(* Logix 5000 AddOnInstructionDefinition export TeNod4TBlocLegal; software revision 28.00 *)

ADD_ON_INSTRUCTION TeNod4TBlocLegal   (* revision 1.1, vendor Scaime *)
VAR_IN_OUT
   Datas : TeNod4TDatas; {required}
END_VAR
VAR_INPUT
   CaptureRead : BOOL; {visible}
   CaptureOnly : BOOL; {visible}
   RequestedID : DINT; {visible}
   Read : BOOL; {visible}
END_VAR
VAR_OUTPUT
   InProgress : BOOL; {visible}
   Done : BOOL; {visible}
   Error : BOOL; {visible}
   CapturedID : DINT; {access Read Only, visible}
END_VAR
VAR
   IntCapture1 : BOOL; {access None}
   IntCapture2 : BOOL; {access None}
   IntCapture3 : BOOL; {access None}
   ReadSeq : BOOL; {access None}
   ReadSeq1 : BOOL; {access None}
   ReadSeq2 : BOOL; {access None}
   ReadSeq3 : BOOL; {access None}
   ReadSeqDone : BOOL; {access None}
   IntRead1 : BOOL; {access None}
END_VAR

ROUTINE Logic   (* ladder *)
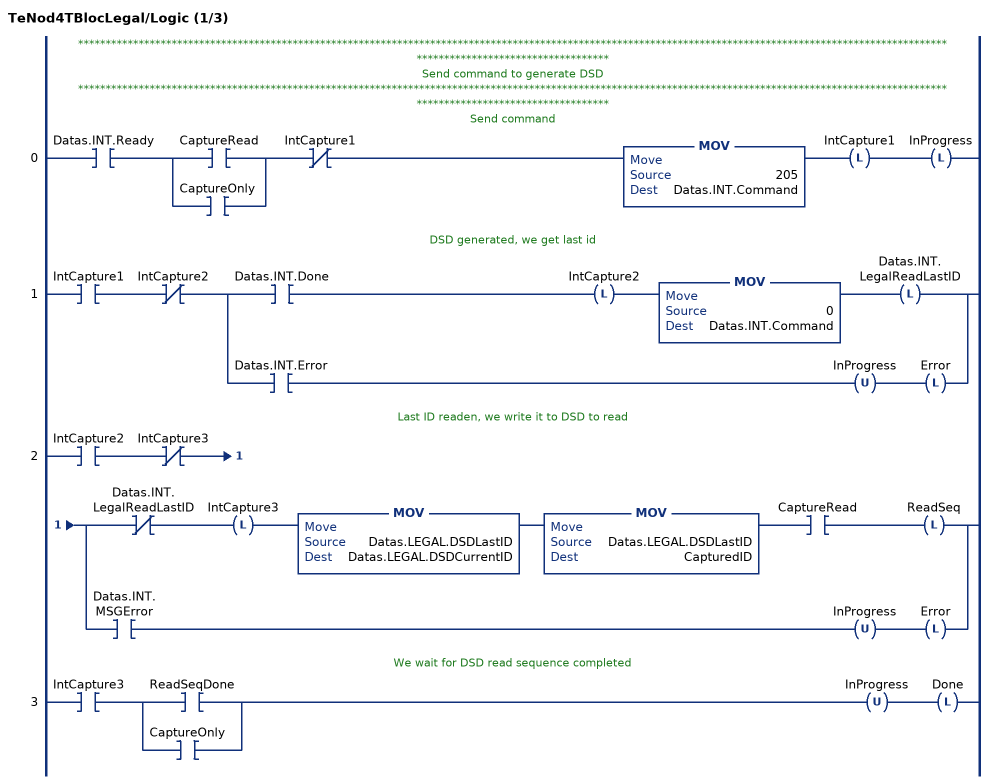
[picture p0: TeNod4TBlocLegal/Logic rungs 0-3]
   // *************************************************************************************************************************************************************************************************
   // Send command to generate DSD
   // *************************************************************************************************************************************************************************************************
   // Send command
   0: XIC(Datas.INT.Ready)[XIC(CaptureRead) ,XIC(CaptureOnly) ]XIO(IntCapture1)MOV(205,Datas.INT.Command)OTL(IntCapture1)OTL(InProgress);
   // DSD generated, we get last id
   1: XIC(IntCapture1)XIO(IntCapture2)[XIC(Datas.INT.Done) OTL(IntCapture2) MOV(0,Datas.INT.Command) OTL(Datas.INT.LegalReadLastID) ,XIC(Datas.INT.Error) OTU(InProgress) OTL(Error) ];
   // Last ID readen, we write it to DSD to read
   2: XIC(IntCapture2)XIO(IntCapture3)[XIO(Datas.INT.LegalReadLastID) OTL(IntCapture3) MOV(Datas.LEGAL.DSDLastID,Datas.LEGAL.DSDCurrentID) MOV(Datas.LEGAL.DSDLastID,CapturedID) XIC(CaptureRead) OTL(ReadSeq) ,XIC(Datas.INT.MSGError) OTU(InProgress) OTL(Error) ];
   // We wait for DSD read sequence completed
   3: XIC(IntCapture3)[XIC(ReadSeqDone) ,XIC(CaptureOnly) ]OTU(InProgress)OTL(Done);
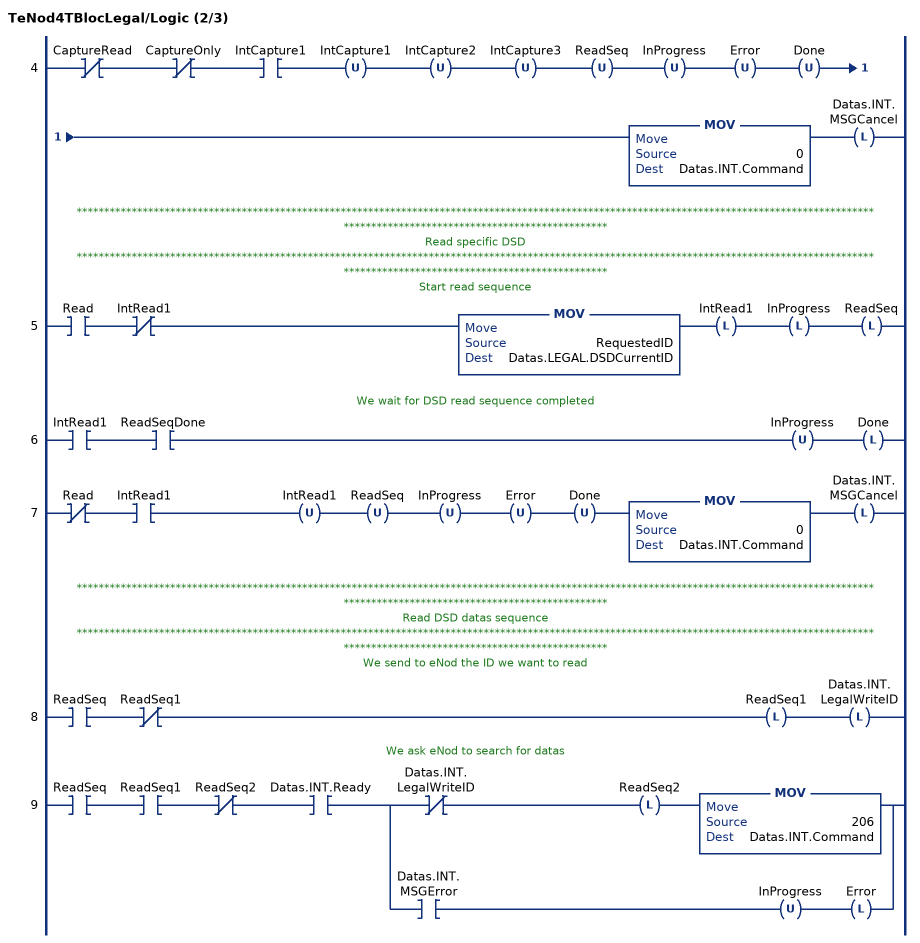
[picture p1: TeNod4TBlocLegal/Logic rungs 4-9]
   4: XIO(CaptureRead)XIO(CaptureOnly)XIC(IntCapture1)OTU(IntCapture1)OTU(IntCapture2)OTU(IntCapture3)OTU(ReadSeq)OTU(InProgress)OTU(Error)OTU(Done)MOV(0,Datas.INT.Command)OTL(Datas.INT.MSGCancel);
   // *************************************************************************************************************************************************************************************************
   // Read specific DSD
   // *************************************************************************************************************************************************************************************************
   // Start read sequence
   5: XIC(Read)XIO(IntRead1)MOV(RequestedID,Datas.LEGAL.DSDCurrentID)OTL(IntRead1)OTL(InProgress)OTL(ReadSeq);
   // We wait for DSD read sequence completed
   6: XIC(IntRead1)XIC(ReadSeqDone)OTU(InProgress)OTL(Done);
   7: XIO(Read)XIC(IntRead1)OTU(IntRead1)OTU(ReadSeq)OTU(InProgress)OTU(Error)OTU(Done)MOV(0,Datas.INT.Command)OTL(Datas.INT.MSGCancel);
   // *************************************************************************************************************************************************************************************************
   // Read DSD datas sequence
   // *************************************************************************************************************************************************************************************************
   // We send to eNod the ID we want to read
   8: XIC(ReadSeq)XIO(ReadSeq1)OTL(ReadSeq1)OTL(Datas.INT.LegalWriteID);
   // We ask eNod to search for datas
   9: XIC(ReadSeq)XIC(ReadSeq1)XIO(ReadSeq2)XIC(Datas.INT.Ready)[XIO(Datas.INT.LegalWriteID) OTL(ReadSeq2) MOV(206,Datas.INT.Command) ,XIC(Datas.INT.MSGError) OTU(InProgress) OTL(Error) ];
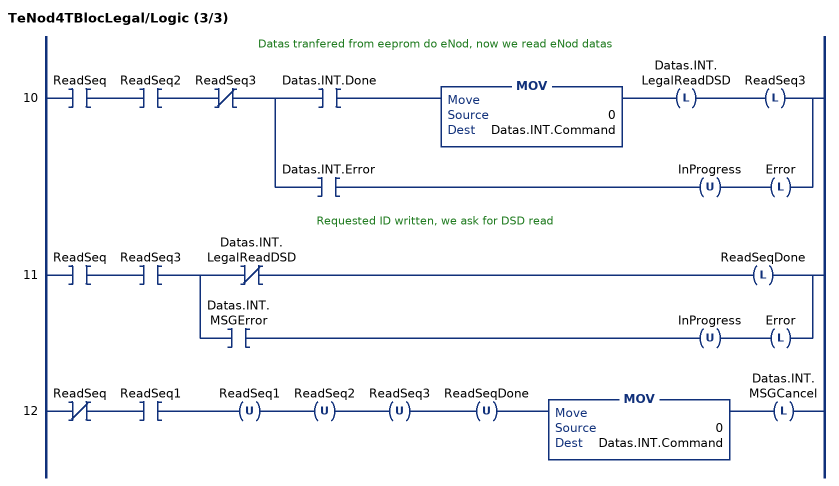
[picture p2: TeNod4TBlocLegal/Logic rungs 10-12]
   // Datas tranfered from eeprom do eNod, now we read eNod datas
   10: XIC(ReadSeq)XIC(ReadSeq2)XIO(ReadSeq3)[XIC(Datas.INT.Done) MOV(0,Datas.INT.Command) OTL(Datas.INT.LegalReadDSD) OTL(ReadSeq3) ,XIC(Datas.INT.Error) OTU(InProgress) OTL(Error) ];
   // Requested ID written, we ask for DSD read
   11: XIC(ReadSeq)XIC(ReadSeq3)[XIO(Datas.INT.LegalReadDSD) OTL(ReadSeqDone) ,XIC(Datas.INT.MSGError) OTU(InProgress) OTL(Error) ];
   12: XIO(ReadSeq)XIC(ReadSeq1)OTU(ReadSeq1)OTU(ReadSeq2)OTU(ReadSeq3)OTU(ReadSeqDone)MOV(0,Datas.INT.Command)OTL(Datas.INT.MSGCancel);
END_ROUTINE
END_ADD_ON_INSTRUCTION
